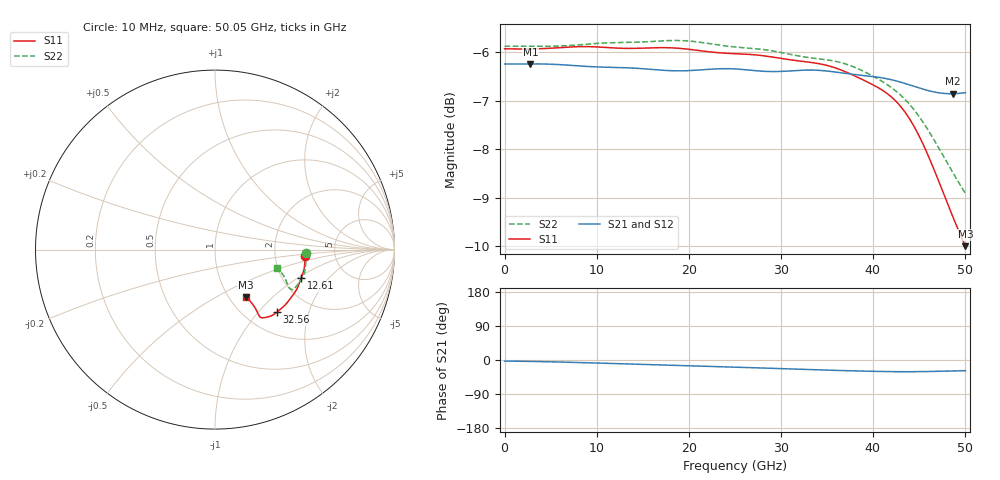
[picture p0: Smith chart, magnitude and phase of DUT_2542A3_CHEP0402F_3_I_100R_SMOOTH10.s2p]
! Touchstone file from project
! Exported from ElectronicsDesktop 2025.1.3
# GHz S MA R 50.000000
! Terminal data exported
! Port[1] = Port1
! Port[2] = Port2
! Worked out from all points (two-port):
!   144 points, 10 MHz to 50.05 GHz, reference 50 ohm
!   highest |S21| = -6.24 dB at 2.81 GHz (marker M1); lowest = -6.9 dB at 48.65 GHz (marker M2)
!   |S21| within 3 dB of the highest: start of sweep to end of sweep
!   lowest |S11| = -10.0 dB at 50.05 GHz (marker M3), VSWR 1.92, Z = 59.5 - j35.1 ohm
!   |S11| at or under -10 dB: 50.04975 GHz to end of sweep
!   |S22| runs from -8.9 to -5.8 dB; largest |S21 - S12| = 0.0039
!   S11 on the Smith chart (normalised r, x): 10 MHz: 3.01, -0.29; 12.61 GHz: 2.53, -1.07; 32.56 GHz: 1.37, -1.26; 50.05 GHz: 1.19, -0.70
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0.01  0.5053 -4.1  0.4873 -2.8  0.4869 -2.4  0.5083 -2.2
! Gamma 0 0 0 0
! Port Impedance 50 0 50 0
2.8096  0.5051 -6.2  0.4875 -3.7  0.4868 -3.4  0.5083 -3.7
4.9093  0.5059 -8.3  0.4872 -4.7  0.4863 -4.5  0.5083 -5.2
8.4088  0.5079 -12.5  0.4849 -6.9  0.4839 -6.8  0.5103 -8.0
12.6082  0.5059 -18.1  0.4833 -9.8  0.4824 -9.7  0.5129 -10.7
16.8076  0.5067 -24.0  0.4804 -12.8  0.4799 -12.7  0.5147 -13.8
20.3071  0.5043 -28.7  0.4799 -15.3  0.4797 -15.1  0.5144 -16.1
23.1067  0.5007 -32.8  0.4818 -17.4  0.4817 -17.2  0.51 -18.1
25.2064  0.4994 -35.8  0.4816 -19.0  0.4814 -18.8  0.5073 -19.8
29.05585  0.4955 -40.4  0.4787 -21.9  0.4785 -21.7  0.5029 -22.1
32.55535  0.4902 -45.5  0.4803 -24.7  0.48 -24.6  0.4956 -24.9
33.6052  0.4887 -47.0  0.4803 -25.6  0.4799 -25.5  0.4941 -25.8
35.35495  0.4848 -49.3  0.4789 -27.0  0.4783 -26.9  0.4917 -26.8
37.45465  0.4765 -52.0  0.4761 -28.4  0.4754 -28.3  0.486 -27.4
40.25425  0.4626 -55.3  0.4727 -30.0  0.4723 -29.8  0.4722 -27.5
42.004  0.4508 -56.3  0.4695 -30.7  0.4694 -30.4  0.4609 -26.9
43.4038  0.436 -56.2  0.4656 -30.9  0.4656 -30.6  0.449 -25.7
44.8036  0.4147 -55.8  0.4611 -30.8  0.4609 -30.4  0.4331 -23.7
46.55335  0.3812 -55.4  0.4562 -30.1  0.456 -29.7  0.4084 -20.8
47.6032  0.36 -55.5  0.4546 -29.6  0.4542 -29.1  0.3925 -19.3
48.65305  0.3397 -56.0  0.4542 -28.9  0.4536 -28.5  0.377 -18.0
50.05285  0.3162 -57.1  0.4553 -28.1  0.4546 -27.7  0.3585 -16.8
